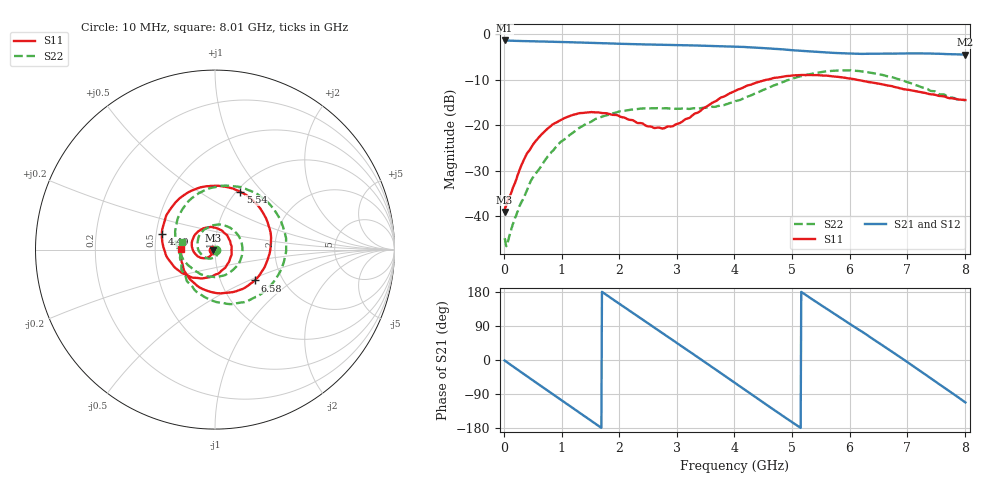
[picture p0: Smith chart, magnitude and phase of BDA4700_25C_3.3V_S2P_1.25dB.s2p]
!Agilent Technologies,E5071B,MY42404982,A.09.10
!Date: Mon Oct 20 18:03:29 2025
!Data & Calibration Information:
!Freq	S11:SOLT2(ON)	S21:SOLT2(ON)	S12:SOLT2(ON)	S22:SOLT2(ON)
# Hz S RI R 50
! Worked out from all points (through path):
!   801 points, 10 MHz to 8.01 GHz, reference 50 ohm
!   highest |S21| = -1.37 dB at 10 MHz (marker M1); lowest = -4.5 dB at 8.01 GHz (marker M2)
!   group delay of S21, straight-line fit = 287 ps
!   lowest |S11| = -39.1 dB at 10 MHz (marker M3), VSWR 1.02, Z = 48.9 - j0.206 ohm
!   |S11| at or under -10 dB: start of sweep to 4.568 GHz; 6.119 GHz to end of sweep
!   |S22| runs from -46.6 to -7.9 dB; largest |S21 - S12| = 0.0097
!   S11 on the Smith chart (normalised r, x): 10 MHz: 0.98, -0.00; 4.49 GHz: 0.54, +0.10; 5.54 GHz: 1.04, +0.77; 6.58 GHz: 1.45, -0.54; 8.01 GHz: 0.68, +0.00
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1e7  -0.0109 -0.00211  0.8538 -0.0184  0.8535 -0.0191  0.00562 -0.000964
3.7e8  -0.0269 -0.0361  0.6452 -0.5377  0.6447 -0.5376  0.015 -0.00884
7.2e8  -0.0736 -0.0469  0.1875 -0.8083  0.1875 -0.8082  -0.000247 -0.0419
1.02e9  -0.1156 -0.0166  -0.2619 -0.7775  -0.2619 -0.7779  -0.0493 -0.0463
1.35e9  -0.1271 0.0475  -0.6498 -0.4828  -0.65 -0.4828  -0.0959 0.0107
1.92e9  -0.0335 0.1252  -0.7256 0.3094  -0.7259 0.3094  -0.00727 0.1362
2.32e9  0.0533 0.091  -0.3334 0.7002  -0.3335 0.7  0.117 0.0947
2.68e9  0.0925 0.016  0.1569 0.7508  0.1556 0.7503  0.1511 -0.027
3.06e9  0.0705 -0.0791  0.5925 0.4732  0.5875 0.4772  0.0773 -0.1302
3.36e9  0.00872 -0.1367  0.7442 0.1002  0.7449 0.1002  -0.0135 -0.1514
3.67e9  -0.0902 -0.1587  0.6744 -0.3103  0.6743 -0.3127  -0.0993 -0.1246
4.01e9  -0.21 -0.1116  0.3599 -0.6368  0.3613 -0.6357  -0.171 -0.063
4.49e9  -0.2957 0.0854  -0.252 -0.6572  -0.252 -0.6593  -0.2222 0.0975
4.92e9  -0.1968 0.2864  -0.6156 -0.2763  -0.6141 -0.2802  -0.1367 0.2802
5.35e9  0.0344 0.3538  -0.6066 0.2168  -0.6079 0.2134  0.1017 0.3529
5.54e9  0.1415 0.3216  -0.4932 0.3951  -0.4944 0.3939  0.2198 0.3173
6.06e9  0.3112 0.0847  0.00396 0.6102  0.00253 0.6133  0.396 0.0369
6.58e9  0.2209 -0.172  0.483 0.3743  0.4843 0.3725  0.2532 -0.2502
6.68e9  0.179 -0.2044  0.5416 0.2827  0.5434 0.2819  0.1999 -0.2773
7.23e9  -0.0653 -0.2213  0.5361 -0.3024  0.536 -0.3029  -0.075 -0.2533
7.62e9  -0.1711 -0.1184  0.2016 -0.573  0.2009 -0.5738  -0.184 -0.1168
8.01e9  -0.1888 0.00284  -0.2232 -0.5529  -0.2213 -0.554  -0.1832 0.0423
